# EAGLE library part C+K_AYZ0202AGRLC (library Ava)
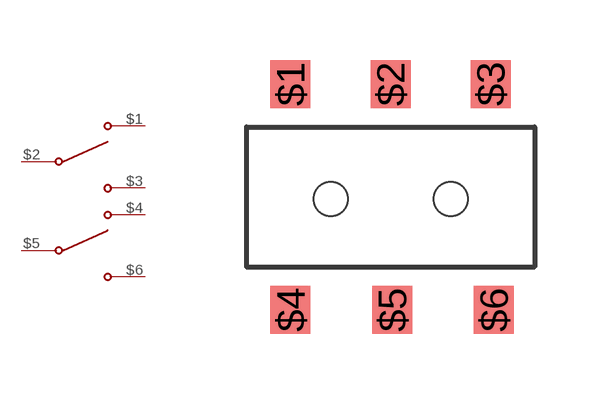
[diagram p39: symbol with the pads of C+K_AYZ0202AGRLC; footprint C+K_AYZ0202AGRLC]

Designator prefix -

## C+K_AYZ0202AGRLC  [C+K_AYZ0202AGRLC]
$1  1
$2  2
$3  3
$4  4
$5  5
$6  6

## Footprint C+K_AYZ0202AGRLC (pad centres in mm)
AYZ0202AGRLC
smd 1 x 1.2: $1 -2.5,2.825; $2 0,2.825; $3 2.5,2.825; $4 -2.5,-2.825; $5 0.04,-2.825; $6 2.58,-2.825
hole 0.85 at -1.5,-0.06
hole 0.85 at 1.5,-0.06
